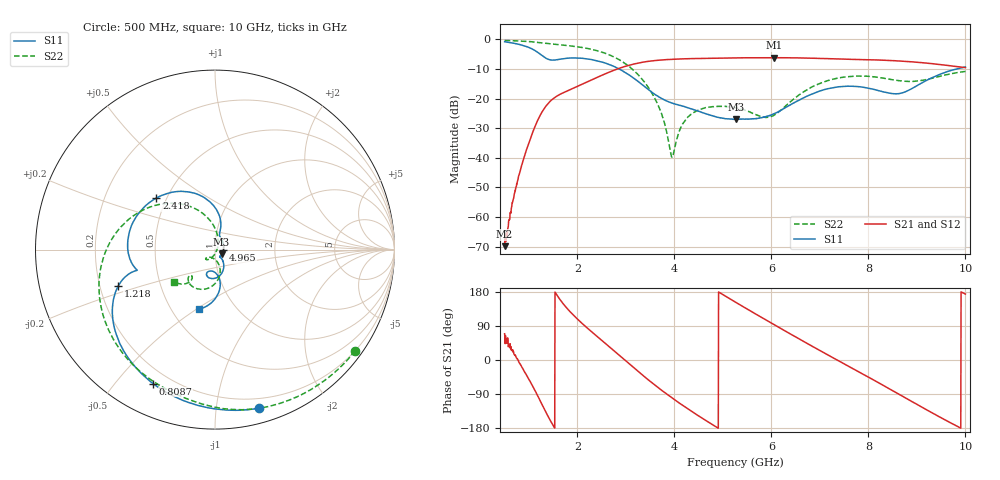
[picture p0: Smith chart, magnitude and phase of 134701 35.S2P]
!  2-Port S-parameters saved by WinCal
! VAR MeasName=S-Parameters (CALIBRATED_DATA) read from VNA (N5242A)
! VAR MeasDate=2013-7-3 16:36:40
! VAR NAME=134701 35
! VAR FILENAME=134701 35.S2P
! VAR DATE=2013-7-3 16:36:40
! VAR PHYS_PORTS=1,2
# Hz S MA R 50
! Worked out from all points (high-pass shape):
!   1601 points, 500 MHz to 10 GHz, reference 50 ohm
!   highest |S21| = -6.14 dB at 6.052 GHz (marker M1); lowest = -69.8 dB at 500 MHz (marker M2)
!   |S21| within 3 dB of the highest: 2.974 GHz to 9.82 GHz (6.846 GHz wide, 107 % of centre)
!   lowest |S11| = -27.0 dB at 5.28 GHz (marker M3), VSWR 1.09, Z = 53.8 - j2.72 ohm
!   |S11| at or under -10 dB: 2.865 GHz to 9.805 GHz (6.94 GHz wide, 110 % of centre)
!   |S22| runs from -39.8 to -0.3 dB; largest |S21 - S12| = 0.0019
!   S11 on the Smith chart (normalised r, x): 500 MHz: 0.12, -1.30; 808.8 MHz: 0.14, -0.63; 1.218 GHz: 0.28, -0.17; 2.418 GHz: 0.44, +0.31; 4.965 GHz: 1.10, -0.01; 10 GHz: 0.68, -0.51
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5e8  0.9175 -74.6  0.0003227 69.3  0.000198 49.0  0.9629 -35.9
6.425e8  0.879 -93.8  0.001469 28.0  0.001445 23.5  0.9545 -46.0
8.0875e8  0.8226 -114.9  0.005515 -8.4  0.005503 -9.1  0.9426 -57.8
1.016562e9  0.724 -139.5  0.01957 -54.7  0.0196 -54.9  0.9205 -72.6
1.218438e9  0.577 -159.3  0.04959 -103.7  0.04948 -104.0  0.8871 -86.9
1.509375e9  0.4485 -165.3  0.1014 -174.6  0.1012 -174.9  0.832 -106.0
2.085312e9  0.483 162.9  0.1735 98.0  0.1727 97.9  0.7351 -145.6
2.417812e9  0.4352 138.7  0.2308 61.0  0.2297 61.1  0.6428 -171.4
2.987812e9  0.2769 97.9  0.3517 -1.4  0.3511 -1.2  0.3913 139.6
3.670625e9  0.1088 74.6  0.4467 -73.5  0.446 -73.4  0.07586 78.9
3.955625e9  0.08419 72.6  0.4626 -100.5  0.4624 -100.5  0.0102 -22.0
4.127812e9  0.07677 68.2  0.4689 -115.8  0.4683 -115.8  0.03194 -100.8
4.294062e9  0.06963 59.7  0.4736 -130.3  0.4738 -130.2  0.05046 -113.3
4.965e9  0.04729 -3.2  0.4858 175.3  0.4862 175.4  0.07411 -133.4
5.25e9  0.04479 -32.5  0.4886 153.4  0.4891 153.4  0.07078 -136.0
5.279688e9  0.04468 -34.4  0.4892 151.2  0.4892 151.1  0.06983 -136.2
6.051562e9  0.05605 -54.8  0.493 93.6  0.4923 93.7  0.05241 -94.1
6.835312e9  0.1195 -67.2  0.4832 36.7  0.4836 36.7  0.1577 -82.0
7.565625e9  0.1623 -95.9  0.4642 -14.8  0.4646 -14.8  0.2345 -109.6
8.420625e9  0.1245 -105.2  0.4428 -75.2  0.4418 -75.3  0.2145 -133.9
9.269688e9  0.2176 -82.8  0.3931 -136.2  0.3942 -136.3  0.2176 -127.8
1e10  0.3434 -104.8  0.3353 174.0  0.3357 174.0  0.2885 -141.7
